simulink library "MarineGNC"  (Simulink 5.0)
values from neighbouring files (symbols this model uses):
  D = 6.533    [RRDcontainer.m]    (also in ExObsCtr.m = sqrt(g/L)*T*Dbis*Tinv)
  delta_max = 20    [RRDcontainer.m]
  G = Hmtrx(r_g)' * G_CG * Hmtrx(r_g)    [Gmtrx.m]    (also in ExLQR.m = -K; ExRRD1.m = [ 0 0.0000704  0; ExRRD2.m = [ 0 0.0000704  0)
  M = 1    [ExWindForce.m]    (also in ExRRD1.m = [ 0.01497    0.0003525     -0.0002205; ExRRD2.m = [ 0.01497    0.0003525     -0.0002205; ExObsCtr.m = T*Mbis*Tinv)
  pathlength = pathlength + sqrt( (xpath(j+1)-xpath(j))^2 + (ypath(j+1)-ypath(j))^2)    [order5.m]    (also in order3.m)
  table = table'    [order5.m]    (also in order3.m)
undefined symbols (not defined in the file or in its folder): Acc, feval, K_supply, rate_max, T_supply
libraries: MarineGNC x24, simulink x18
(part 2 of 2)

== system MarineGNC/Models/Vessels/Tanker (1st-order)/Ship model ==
  note: heading angle
  rudder angle : Inport
  " Nomoto  time constant" : Gain  Gain=1/T_supply
  Integrator : Integrator
  Integrator1 : Integrator
  Nomoto gain constant : Gain  Gain=K_supply
  Sum : Sum  Inputs=|+-
  heading angle : Outport
  heading rate : Outport  Port=2
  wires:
  " Nomoto  time constant"/1 -> Integrator/1
  Sum/1 -> " Nomoto  time constant"/1
  rudder angle/1 -> Nomoto gain constant/1
  Nomoto gain constant/1 -> Sum/1
  Integrator/1 -> heading rate/1, Integrator1/1, Sum/2  "heading  rate"
  Integrator1/1 -> heading angle/1

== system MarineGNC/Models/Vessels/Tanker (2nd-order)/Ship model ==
  note: heading angle
  rudder angle : Inport
  Integrator : Integrator
  Nomoto 2nd-order model : TransferFcn  Numerator=[K*T3 K]  Denominator=[T1*T2 (T1+T2) 1]
  heading angle : Outport
  heading rate : Outport  Port=2
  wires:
  Integrator/1 -> heading angle/1
  Nomoto 2nd-order model/1 -> Integrator/1, heading rate/1  "heading rate"
  rudder angle/1 -> Nomoto 2nd-order model/1
